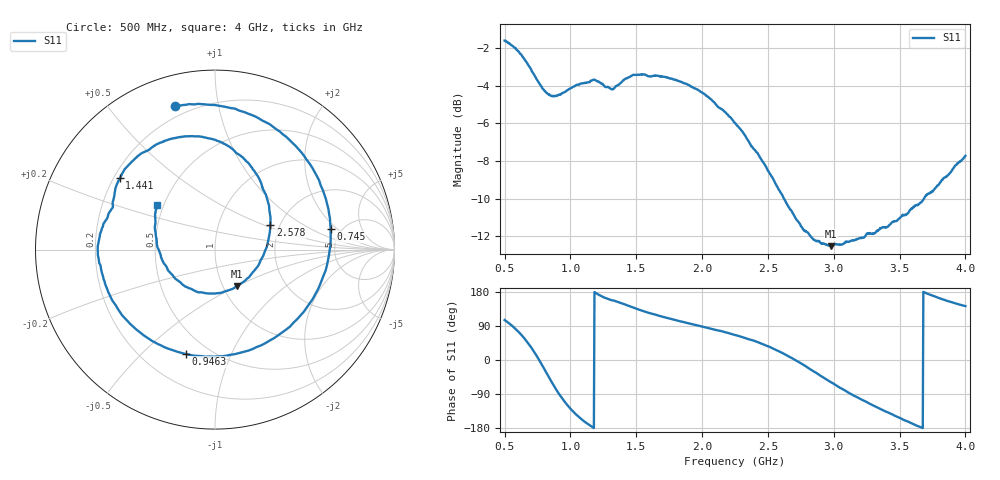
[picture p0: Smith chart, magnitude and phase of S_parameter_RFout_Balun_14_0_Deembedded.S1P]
!Agilent Technologies,E5071B,MY42403504,A.06.51
!Date: Wed Feb 26 14:58:04 2014
!Data & Calibration Information:
!Freq	S11:SOLT1(ON)
# Hz S dB R 50
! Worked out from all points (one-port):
!   801 points, 500 MHz to 4 GHz, reference 50 ohm
!   lowest |S11| = -12.5 dB at 2.981 GHz (marker M1), VSWR 1.62, Z = 58.2 - j25 ohm
!   |S11| at or under -10 dB: 2.622 GHz to 3.685 GHz (1.062 GHz wide, 33.7 % of centre)
!   S11 on the Smith chart (normalised r, x): 500 MHz: 0.15, +0.75; 745 MHz: 4.08, +1.65; 946.2 MHz: 0.38, -0.69; 1.441 GHz: 0.22, +0.32; 2.578 GHz: 1.78, +0.55; 4 GHz: 0.46, +0.28
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5e8  -1.61 105.5
5.7e8  -1.96 86.1
6.26875e8  -2.36 66.5
6.925e8  -3.05 38.0
7.45e8  -3.68 10.2
7.93125e8  -4.20 -18.6
8.5e8  -4.54 -53.7
8.9375e8  -4.54 -79.1
9.375e8  -4.40 -101.6
9.4625e8  -4.38 -105.8
1.025e9  -4.06 -137.7
1.108125e9  -3.86 -163.0
1.17375e9  -3.70 -178.6
1.235e9  -3.90 168.5
1.375e9  -3.91 151.6
1.440625e9  -3.57 143.2
1.571875e9  -3.43 126.5
1.8125e9  -3.74 104.0
2.018125e9  -4.46 86.5
2.25e9  -5.98 66.0
2.578125e9  -9.45 23.8
2.6875e9  -10.76 3.7
2.980625e9  -12.52 -58.8
3.125e9  -12.26 -88.6
3.34375e9  -11.64 -127.1
3.5625e9  -10.78 -162.4
3.71125e9  -9.76 174.9
4e9  -7.73 142.3
